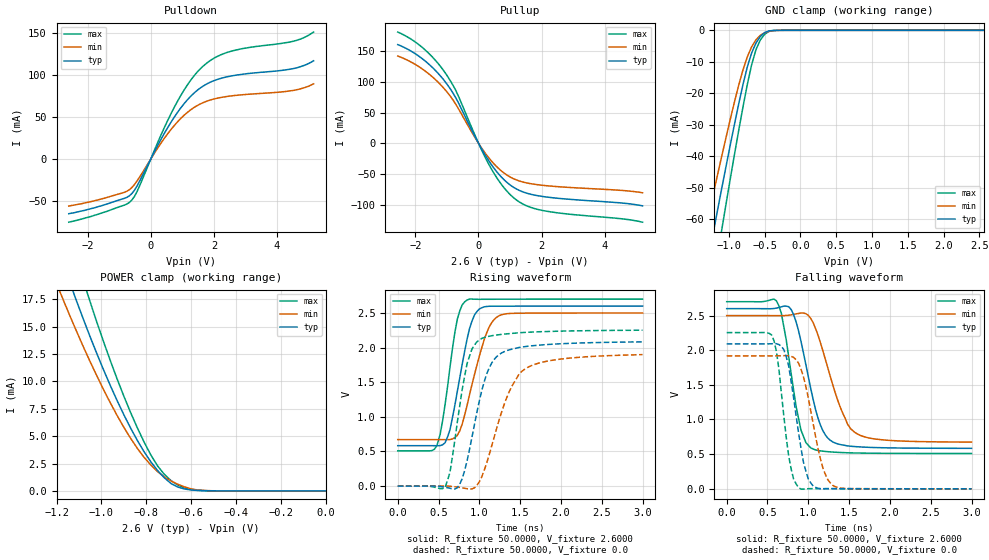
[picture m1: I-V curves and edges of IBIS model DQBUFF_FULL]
| IBIS file mic_t27b.ibs created by s2ibis3 verion 1.1
| North Carolina State University, ERL, 2006
[IBIS ver] 4.1
[File name] mic_t27b_dq_bird95.ibs
[File Rev] 0.1
[Date]  28 mar 2006
[Source] IBIS macro task group conversion of Micron HSPICE model
   http://micron.com/products/dram/ddrsdram/part.aspx
   Select part MT46V32M16TG-5B
   Download HSPICE models and use as a basis:
   512meg_ddr400_spice/t27b_ddr400_spice/t27b_ddr400_dq.sp
[Notes]
   !!! THIS FILE IS NOT IBIS COMPLIANT !!!
  It contains [Composite Current] data specified by BIRD95, which is
  not incorporated into any approved IBIS specification. This data was
  produced using s2ibis3 and a PERL script that runs additional simulations
  and creates the data files.
  About the buffer:
  o The HSPICE model for the Micron t27b DQ buffer is modeled.
  o This is a 2.6V buffer, not 2.5V
  o The buffer is configured for full strength operation.
  28 mar 2006 Mike LaBonte
   Created this IBIS file using s2ibis3. Wrote PERL script to run
   simulations measuring VCCS2I current and extract data. Added
   [Composite Current] data to IBIS file.
|   Component MIC_DDR_SDRAM_T27B_DQBUFF
[Component] MIC_DDR_SDRAM_T27B_DQBUFF
[Manufacturer] Micron Technology
[Package]
| variable   typ   min   max
R_pkg   0.4800   20.0000m   0.9300
L_pkg   3.1200nH   0.5200nH   5.7100nH
C_pkg   1.6300pF   0.5300pF   2.7200pF
[Pin]  signal_name   model_name   R_pin   L_pin   C_pin
vccq   vccq   POWER
vssq   vssq   GND
|ena   ena   dummy
|in   in   dummy
DQ   DQ   DQBUFF_FULL
| Models and submodels in the file (1): DQBUFF_FULL (I/O)
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|   Model DQBUFF_FULL
[Model]  DQBUFF_FULL
Model_type I/O
Polarity   Non-Inverting
Enable   Active-High
Vinl =   0.9900V
Vinh =   1.6100V
Vmeas =  1.3000V
Cref =   30.0000pF
Rref =   50.0000
Vref =   1.3000V
C_comp   1.1000pF   1.1000pF   1.1000pF
[Temperature Range]   40.0000   85.0000   0.0
[Voltage Range]   2.6000V   2.5000V   2.7000V
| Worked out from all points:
|   slope of the pulldown table from 0 to 0.39 V, typ, clamps not added: 14 ohm
|   slope of the pullup table from 0 to 0.39 V, typ, clamps not added: 11.7 ohm
|   GND clamp passes 1 mA (typ) near -0.51 V on its own axis
|   POWER clamp passes 1 mA (typ) near -0.71 V on its own axis
|   rising waveform, R_fixture 50.0000, V_fixture 2.6000: 20-80 % time 195ps typ, 243ps min, 156ps max; typ from 0.583 V to 2.6 V
|   rising waveform, R_fixture 50.0000, V_fixture 0.0: 20-80 % time 248ps typ, 336ps min, 185ps max; typ from 0 V to 2.08 V
|   falling waveform, R_fixture 50.0000, V_fixture 2.6000: 20-80 % time 232ps typ, 302ps min, 181ps max; typ from 2.6 V to 0.584 V
|   falling waveform, R_fixture 50.0000, V_fixture 0.0: 20-80 % time 162ps typ, 202ps min, 132ps max; typ from 2.09 V to 0 V
[Pulldown]
|Voltage   I(typ)   I(min)   I(max)
-2.6V     -65.2mA    -56.1mA    -75.3mA
-920mV    -47.87mA   -40.67mA   -55.99mA
-600mV    -41.11mA   -34.05mA   -48.9mA
-440mV    -32.42mA   -26.4mA    -39.12mA
360mV     25.9mA     20.94mA    31.7mA
840mV     55.15mA    43.94mA    68.32mA
1.32V     76.76mA    60.07mA    96.62mA
1.8V      89.92mA    69.21mA    115mA
2.52V     98.69mA    75.02mA    128.1mA
4.44V     107.1mA    81.31mA    139.6mA
4.76V     110.2mA    83.73mA    143.1mA
5.16V     117mA      89.5mA     151.2mA
[Pullup]
|Voltage   I(typ)   I(min)   I(max)
-2.56V    160.5mA    142mA      180.9mA
-1.76V    136.7mA    120.1mA    155mA
-1.36V    118.1mA    103.3mA    134.6mA
-1.04V    98.99mA    86.01mA    113.5mA
-720mV    73.92mA    63.46mA    86mA
0V        1.715nA    1.39nA     2.124nA
400mV     -34.15mA   -28.32mA   -41.04mA
800mV     -58.94mA   -48.13mA   -71.89mA
1.2V      -74.37mA   -59.72mA   -92.24mA
1.6V      -82.3mA    -65.33mA   -103.4mA
2.08V     -87mA      -68.72mA   -109.9mA
5.2V      -101.9mA   -80.7mA    -128.5mA
[GND_clamp]
|Voltage   I(typ)   I(min)   I(max)
-2.6V     -243.6mA   -206.1mA   -287.5mA
-1.34V    -79.39mA   -64.85mA   -97.71mA
-1.28V    -72.04mA   -58.59mA   -89.08mA
-1.22V    -64.76mA   -52.4mA    -80.52mA
-1.16V    -57.57mA   -46.27mA   -72.05mA
-1.1V     -50.47mA   -40.21mA   -63.7mA
-1.04V    -43.47mA   -34.24mA   -55.46mA
-860mV    -23.27mA   -17.33mA   -31.67mA
-740mV    -11.55mA   -8.364mA   -17.1mA
-620mV    -4.025mA   -3.002mA   -6.134mA
-500mV    -726.8uA   -782uA     -1.266mA
2.56V     849.1pA    14.97nA    323.9pA
[POWER_clamp]
|Voltage   I(typ)   I(min)   I(max)
-2.58V    123.2mA    106.8mA    143.3mA
-1.2V     22.51mA    18.96mA    27.35mA
-1.17V    20.74mA    17.45mA    25.24mA
-1.11V    17.31mA    14.55mA    21.14mA
-1.08V    15.67mA    13.15mA    19.17mA
-1.05V    14.07mA    11.8mA     17.26mA
-960mV    9.615mA    8.037mA    11.89mA
-870mV    5.745mA    4.813mA    7.168mA
-780mV    2.666mA    2.367mA    3.296mA
-690mV    681.1uA    908.7uA    947.2uA
-570mV    39.27uA    84.83uA    59.85uA
0V        862.8pA    14.56nA    349.7pA
[Ramp]
| variable   typ   min   max
dV/dt_r  1.2492/0.2476n   1.1388/0.3362n   1.3500/0.1846n
dV/dt_f  1.2097/0.2318n   1.0958/0.3020n   1.3145/0.1806n
R_load = 50.0000
[Rising Waveform]
R_fixture= 50.0000
V_fixture= 2.6000
V_fixture_min= 2.5000
V_fixture_max= 2.7000
|time   V(typ)   V(min)   V(max)
0s        583.2mV    671.3mV    508.9mV
480ps     582.4mV    671.3mV    585mV
550ps     595.7mV    671mV      944.1mV
640ps     812.2mV    671.6mV    1.714V
730ps     1.365V     731.6mV    2.408V
850ps     2.123V     1.165V     2.687V
940ps     2.469V     1.607V     2.698V
1.06ns    2.588V     2.115V     2.697V
1.24ns    2.597V     2.458V     2.698V
3ns       2.599V     2.499V     2.699V
[Rising Waveform]
R_fixture= 50.0000
V_fixture= 0.0
V_fixture_min= 0.0
V_fixture_max= 0.0
|time   V(typ)   V(min)   V(max)
0s        0V         0V         0V
580ps     -17.05mV   800.6uV    -19.62mV
640ps     -30.96mV   -2.539mV   198.1mV
790ps     106.6mV    -25.44mV   1.395V
910ps     708.2mV    -40.53mV   1.98V
1.03ns    1.381V     135.4mV    2.132V
1.21ns    1.866V     823.6mV    2.181V
1.36ns    1.965V     1.346V     2.2V
1.55ns    2.012V     1.683V     2.218V
3ns       2.082V     1.898V     2.25V
[Falling Waveform]
R_fixture= 50.0000
V_fixture= 2.6000
V_fixture_min= 2.5000
V_fixture_max= 2.7000
|time   V(typ)   V(min)   V(max)
0s        2.6V       2.5V       2.7V
610ps     2.608V     2.499V     2.711V
670ps     2.626V     2.498V     2.531V
820ps     2.514V     2.516V     1.426V
910ps     2.131V     2.537V     849.5mV
1.03ns    1.446V     2.458V     589.8mV
1.21ns    775.7mV    1.865V     538.5mV
1.42ns    631.8mV    1.096V     522.7mV
1.58ns    608.3mV    806.3mV    516.7mV
3ns       583.9mV    673.6mV    509.2mV
[Falling Waveform]
R_fixture= 50.0000
V_fixture= 0.0
V_fixture_min= 0.0
V_fixture_max= 0.0
|time   V(typ)   V(min)   V(max)
0s        2.091V     1.918V     2.254V
550ps     2.093V     1.918V     2.221V
610ps     2.094V     1.918V     1.98V
730ps     1.904V     1.921V     740mV
820ps     1.314V     1.896V     139.9mV
910ps     591.6mV    1.728V     -4.724mV
1.06ns    37.95mV    937.8mV    2.426mV
1.18ns    518.1uV    296.4mV    1.597mV
1.3ns     2.432mV    49.09mV    940.9uV
3ns       92.31uV    134.8uV    70.75uV
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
